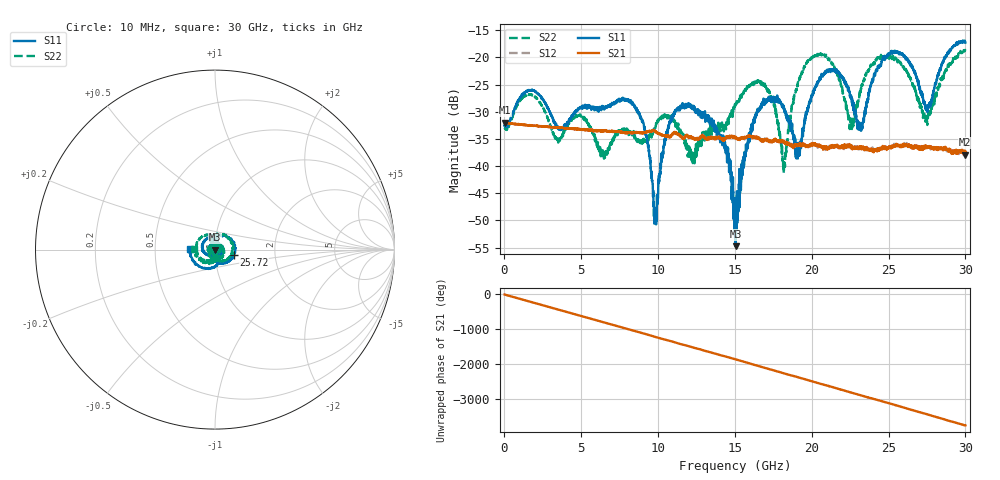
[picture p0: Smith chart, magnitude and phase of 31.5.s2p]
#  HZ  S  DB  R  50.00
! Rohde & Schwarz Vector Network Analyzer
! Rohde-Schwarz,ZNB40-4Port,1311601084101679,3.45
! Created: UTC 10/20/2022, 5:22:05 PM
! freq[Hz]  db:S11  ang:S11  db:S31  ang:S31  db:S13  ang:S13  db:S33  ang:S33
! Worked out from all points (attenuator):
!   3000 points, 10 MHz to 30 GHz, reference 50 ohm
!   highest |S21| = -32.02 dB at 30 MHz (marker M1); lowest = -37.9 dB at 29.95 GHz (marker M2)
!   lowest |S11| = -54.7 dB at 15.04 GHz (marker M3), VSWR 1.00, Z = 49.8 - j0.00343 ohm
!   |S11| at or under -10 dB: start of sweep to end of sweep
!   |S22| runs from -41.4 to -18.6 dB; largest |S21 - S12| = 0.0015
!   S11 on the Smith chart (normalised r, x): 10 MHz: 0.95, +0.00; 25.72 GHz: 1.23, -0.08; 30 GHz: 0.76, +0.01
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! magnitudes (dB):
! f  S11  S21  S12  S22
! 10 MHz  -32.5  -32.0  -32.0  -32.9
! 30 MHz  -32.7  -32.0  -32.0  -33.1
! 5.01 GHz  -29.4  -33.3  -33.3  -30.9
! 6.42 GHz  -29.0  -33.6  -33.6  -37.6
! 8.33 GHz  -28.2  -33.9  -34.0  -34.3
! 10.01 GHz  -43.2  -34.0  -34.1  -31.8
! 10.78 GHz  -31.8  -34.7  -34.5  -31.1
! 12.03 GHz  -28.9  -34.8  -34.7  -36.4
! 14.24 GHz  -34.9  -35.3  -35.1  -32.5
! 15.01 GHz  -53.2  -34.9  -34.9  -28.9
! 15.04 GHz  -54.7  -34.8  -34.8  -28.8
! 16.43 GHz  -30.1  -34.8  -34.8  -24.6
! 18.2 GHz  -29.6  -35.6  -35.5  -39.3
! 19.08 GHz  -37.1  -36.1  -36.3  -24.9
! 20.01 GHz  -27.1  -36.2  -35.9  -19.9
! 22.6 GHz  -28.0  -36.3  -36.5  -33.5
! 23.25 GHz  -32.4  -36.5  -36.6  -25.1
! 25.01 GHz  -19.6  -36.6  -36.5  -20.2
! 25.72 GHz  -19.3  -36.3  -36.3  -20.9
! 27.41 GHz  -29.0  -36.2  -36.5  -31.1
! 29.95 GHz  -17.0  -37.9  -37.7  -18.8
! 30 GHz  -17.3  -37.3  -37.3  -18.7
